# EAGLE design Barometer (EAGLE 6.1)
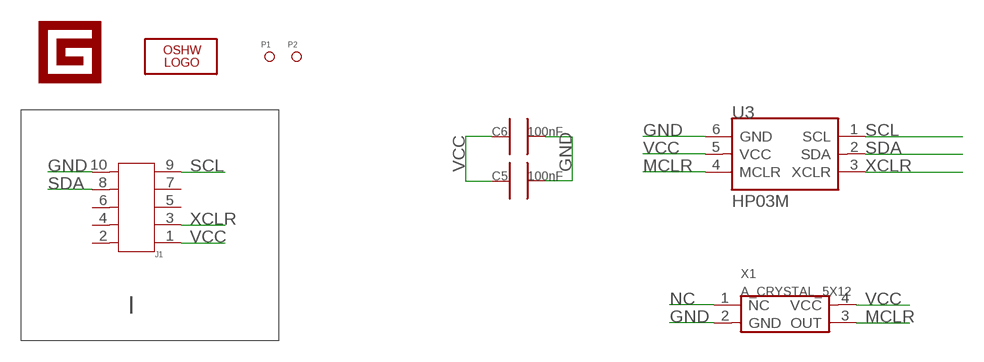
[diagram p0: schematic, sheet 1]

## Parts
C5  100nF  C0603_S  [0603_S]
C6  100nF  C0603_S  [0603_S]
J1  HEADER-SHF-105-01-L-D-SM  [SHF-105-01-L-D-SM]
LOGO1  LOGO-OSHW-FILLX0150-NT  [OSHW_FILLX150_NOTEXT]
P1  PAD-MARK  [ROUND-MARK-0.635]
P2  PAD-MARK  [ROUND-MARK-0.635]
U3  HP03M  [HP03M]
U$1  LOGO-GADGETEER-NORMAL  [GADGETEER-SILK]
X1  A_CRYSTAL_5X12  [4P_5X12]

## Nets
GND: C5.2 C6.2 J1.10 U3.6(GND) X1.2(GND)
MCLR: U3.4(MCLR) X1.3(OUT)
NC: X1.1(NC)
SCL: J1.9 U3.1(SCL)
SDA: J1.8 U3.2(SDA)
VCC: C5.1 C6.1 J1.1 U3.5(VCC) X1.4(VCC)
XCLR: J1.3 U3.3(XCLR)
Unconnected: J1.2 J1.4 J1.5 J1.6 J1.7

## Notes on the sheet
- I

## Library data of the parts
C5 C6 = CPT_SMD:C0603
J1 = Connector:HEADER-SHF-105-01-L-D-SM
LOGO1 = Logo:LOGO-OSHW-FILL
P1 P2 = Discreter:PAD-MARK
U3 = EXT_moudle:HP03M
U$1 = Logo:LOGO-GADGETEER
X1 = CPT_SMD:A_CRYSTAL

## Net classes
0 default: width 0.152 mm, drill 0.305 mm, clearance 0.152 mm

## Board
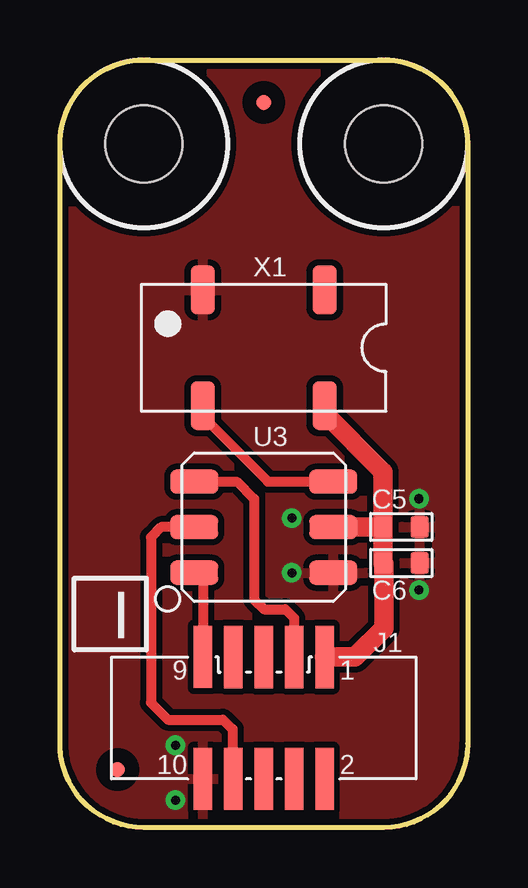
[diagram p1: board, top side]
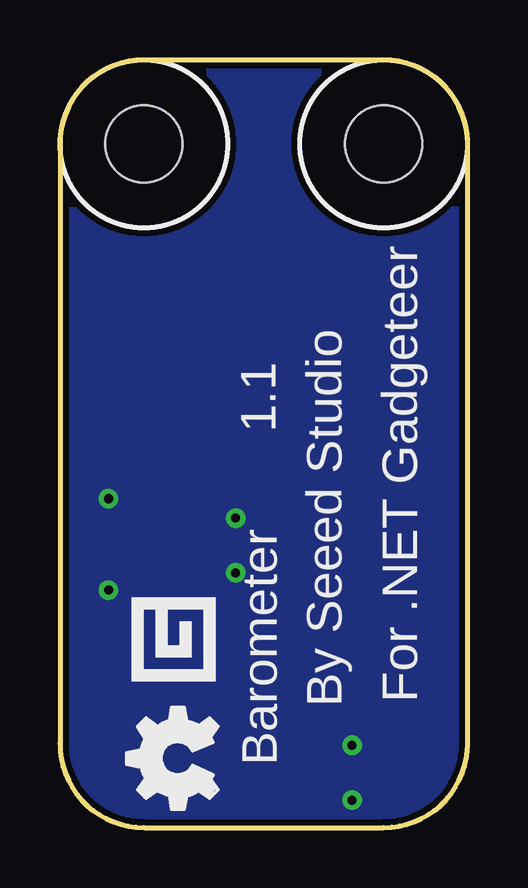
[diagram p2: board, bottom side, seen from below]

Size 17 x 32 mm. Coordinates in mm from the lower left corner, seen from the top.
Outline: 3.5,0 arc-90 0,3.5 0,28.5 arc-90 3.5,32 13.5,32 arc-90 17,28.5 17,3.5 arc-90 13.5,0 3.5,0
Copper layers (1*16): Top 0.035mm / dielectric 1.5mm / Bottom 0.035mm
Design rules: minimum track width 10mil, minimum drill 12mil, track to track 8mil, track to pad 8mil, pad to pad 8mil, via to via 8mil, smd to smd 8mil, copper to edge 10mil, drill to drill 8mil, minimum pad ring 10mil, minimum via ring 8mil, stop-mask expansion 4mil, vias tented up to drill 100mil, thermal gap 10mil

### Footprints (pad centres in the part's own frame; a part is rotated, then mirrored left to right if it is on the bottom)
0603_S = smd 0.762 x 0.889: 1 -0.762,0; 2 0.762,0
SHF-105-01-L-D-SM = smd 0.762 x 2.6: 1 -2.54,-2.54; 2 -2.54,2.54; 3 -1.27,-2.54; 4 -1.27,2.54; 5 0,-2.54; 6 0,2.54; 7 1.27,-2.54; 8 1.27,2.54; 9 2.54,-2.546; 10 2.54,2.54
ROUND-MARK-0.635 = smd 0.635 x 0.635: P$1 0,0
HP03M = smd 2 x 1: 1 2.9,1.9; 2 2.9,0; 3 2.9,-1.9; 4 -2.9,-1.9; 5 -2.9,0; 6 -2.9,1.9
HOLE-D-3.2/7.0 = hole 3.2: 0,0
4P_5X12 = smd 1.016 x 2.032: 1 -2.54,-2.413; 2 2.54,-2.413; 3 2.54,2.413; 4 -2.54,2.413

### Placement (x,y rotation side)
C5  14.24,12.53 0 top
C6  14.24,11.03 0 top
J1  8.5,4.57 180 top
LOGO1  10.4,0.76 90 bottom
P1  8.5,30.22 90 top
P2  2.4,2.41 90 top
U3  8.5,12.53 180 top
U$1  12.69,8.25 90 bottom
U$3  PAD-HOLE'3.2/7.0'  [HOLE-D-3.2/7.0]  3.5,28.5 90 top
U$5  PAD-HOLE'3.2/7.0'  [HOLE-D-3.2/7.0]  13.5,28.5 90 top
X1  8.5,20 180 top

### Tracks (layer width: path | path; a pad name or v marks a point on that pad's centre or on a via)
GND  (via drill 0.38 pad 0.81)
  other vias: 9.67,10.62 9.67,12.91 4.82,1.14 4.82,3.43 14.97,13.71 14.97,9.91
  pour Top (isolate 0.254): -0.39,-0.51 -0.39,32.51 17.39,31.88 17.39,-0.51
  pour Bottom (isolate 0.254): -0.39,-0.51 -0.39,32.51 17.39,31.88 17.39,-0.51
MCLR
  Top 0.406: U3.4 8.68,14.43 6,17.1 6,17.55 X1.3
SCL
  Top 0.406: J1.9 5.96,10.26 U3.1
SDA
  Top 0.406: U3.2 4.22,12.53 3.8,12.1 3.8,5.2 4.5,4.5 6.8,4.5 7.2,4.1 7.2,2.03 J1.8
VCC
  Top 0.813: C5.1 C6.1 13.5,11 13.5,8.3 12.31,7.11 J1.1 | U3.5 C5.1 | C5.1 13.48,14.82 11,17.3 11,17.55 X1.4
XCLR
  Top 0.406: U3.3 5.62,14.4 7.4,14.4 8.1,13.7 8.1,9.5 8.5,9.1 9.4,9.1 9.77,8.73 J1.3

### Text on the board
tPlace: I
bPlace: For .NET Gadgeteer | By Seeed Studio | 1.1 | Barometer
